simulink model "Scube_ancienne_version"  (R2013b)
settings: Solver=ode23t  StartTime=0.0  StopTime=100  RelTol=1e-3
libraries: fl_lib x14, nesl_utility x4, elec_lib x1

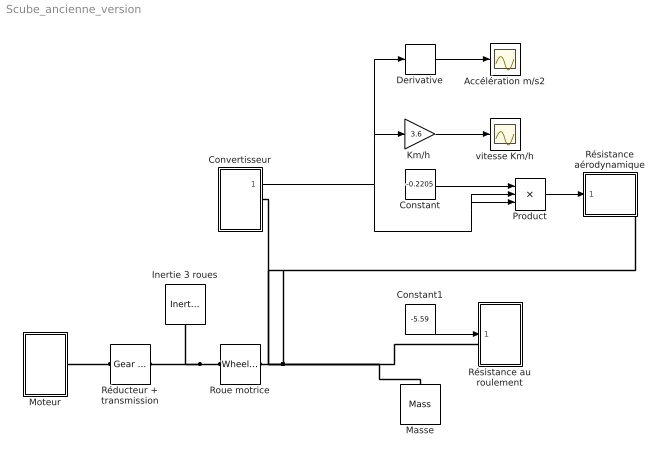
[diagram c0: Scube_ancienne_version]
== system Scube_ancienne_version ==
  Accélération m/s2 : Scope
  Constant : Constant  Value=-0.2205
  Constant1 : Constant  Value=-5.59
  Convertisseur : Subsystem
  Derivative : Derivative
  Inertie 3 roues : fl_lib/Mechanical/Rotational Elements/Inertia  inertia=0.01 kg*m^2  initial_velocity=0 rad/s  t_Log=off  LocalVarNames=|t  LocalVarDescs=|t  LocalVarLogging=0
  "Km/h " : Gain  Gain=3.6
  Masse : fl_lib/Mechanical/Translational Elements/Mass  mass=10 kg  initial_velocity=0 m/s  f_Log=off  LocalVarNames=|f  LocalVarDescs=|f  LocalVarLogging=0
  Moteur : Subsystem
  Product : Product  Inputs=3
  Roue motrice : fl_lib/Mechanical/Mechanisms/Wheel and Axle  R=50 mm  or=1  orient=1  t_Log=off  f_Log=off  LocalVarNames=|t|f  LocalVarDescs=|t|f  LocalVarLogging=[0 0]
  Réducteur + transmission : fl_lib/Mechanical/Mechanisms/Gear Box  ratio=13.84  t_in_Log=off  t_out_Log=off  LocalVarNames=|t_in|t_out  LocalVarDescs=|t_in|t_out  LocalVarLogging=[0 0]
  Résistance au roulement : Subsystem
  Résistance aérodynamique : Subsystem
  vitesse Km/h : Scope
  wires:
  "Km/h "/1 -> vitesse Km/h/1
  Constant1/1 -> Résistance au roulement/1(In1)
  Convertisseur/1(V (m/s)) -> Product/2, Product/3, Derivative/1, "Km/h "/1
  Constant/1 -> Product/1
  Product/1 -> Résistance aérodynamique/1(In1)
  Derivative/1 -> Accélération m/s2/1
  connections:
  Roue motrice/RConn1 -- Résistance aérodynamique/RConn1 -- Convertisseur/RConn1 -- Résistance au roulement/LConn1 -- Masse/LConn1
  Roue motrice/LConn1 -- Inertie 3 roues/LConn1 -- Réducteur + transmission/RConn1
  Moteur/RConn1 -- Réducteur + transmission/LConn1

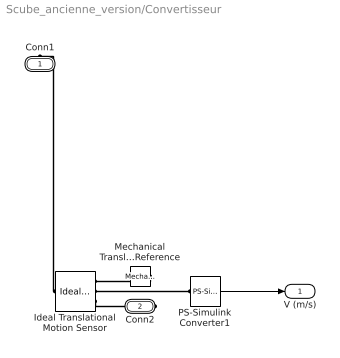
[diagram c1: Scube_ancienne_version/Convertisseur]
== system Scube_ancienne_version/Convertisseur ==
  Ideal Translational Motion Sensor : fl_lib/Mechanical/Mechanical Sensors/Ideal Translational Motion Sensor  offset=0 m  v_Log=off  f_Log=off  x_Log=off  LocalVarNames=|v|f|x  LocalVarDescs=|v|f|x  LocalVarLogging=[0 0 0]
  Mechanical Translational Reference : fl_lib/Mechanical/Translational Elements/Mechanical Translational Reference  f_Log=off  LocalVarNames=|f  LocalVarDescs=|f  LocalVarLogging=0
  PS-Simulink Converter1 : nesl_utility/PS-Simulink Converter  PhysicalDomain=network_engine_domain  SubClassName=ps_output  LeftPortType=input  RightPortType=output  PseudoPeriodic=off  Frequencies=[]  Unit=m/s  AffineConversion=off
  Conn1 : PMIOPort  Port=1  Side=Right
  Conn2 : PMIOPort  Port=2  Side=Right
  V (m/s) : Outport
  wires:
  PS-Simulink Converter1/1 -> V (m/s)/1
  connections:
  Ideal Translational Motion Sensor/RConn3 -- Conn2/RConn1
  Ideal Translational Motion Sensor/LConn1 -- Conn1/RConn1
  Mechanical Translational Reference/LConn1 -- Ideal Translational Motion Sensor/RConn1
  PS-Simulink Converter1/LConn1 -- Ideal Translational Motion Sensor/RConn2

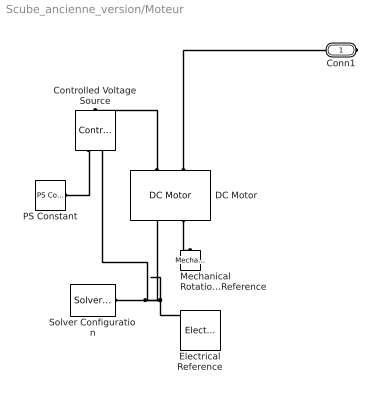
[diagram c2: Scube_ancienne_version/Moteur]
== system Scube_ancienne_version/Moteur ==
  Controlled Voltage Source : fl_lib/Electrical/Electrical Sources/Controlled Voltage Source  i_Log=off  v_Log=off  LocalVarNames=|i|v  LocalVarDescs=|i|v  LocalVarLogging=[0 0]
  DC Motor : elec_lib/Actuators & Drivers/Rotational Actuators/DC Motor  parameterization=2  Ra=2 Ohm  La=1 mH  emf_or_torque=2  Kv=4e-3 V/rpm  Ki=4e-2 N*m/A  T_stall=1.83333 N*m  w_max=3700 rpm  w_rated=3200 rpm  P_rated=600 W  V_rated=48 V  J=0.006 kg*m^2  lam_param=2  lam=0 N*m/(rad/s)  i_noload=2.2 A  V_i_noload=48 V  speed0=0 rpm  current_Log=off  voltage_Log=off  power_Log=off  i2r_Log=off  torque_Log=off  speed_Log=off  LocalVarNames=|current|voltage|power|i2r|torque|speed  LocalVarDescs=|Current (A)|Voltage (V)|Power (W)|Electrical losses (W)|Torque (Nm)|Angular speed (rad/s)  LocalVarLogging=[0 0 0 0 0 0]  alpha=0.00393 1/K  Tmeas=25 C  thermal_mass=100 J/K  initial_temperature=25 C
  Electrical Reference : fl_lib/Electrical/Electrical Elements/Electrical Reference  i_Log=off  LocalVarNames=|i  LocalVarDescs=|i  LocalVarLogging=0
  Mechanical Rotational Reference : fl_lib/Mechanical/Rotational Elements/Mechanical Rotational Reference  t_Log=off  LocalVarNames=|t  LocalVarDescs=|t  LocalVarLogging=0
  PS Constant : fl_lib/Physical Signals/Sources/PS Constant  constant=48  LocalVarLogging=[]
  Solver Configuration : nesl_utility/Solver Configuration  PhysicalDomain=network_engine_domain  SubClassName=solver  LeftPortType=input  RightPortType=generic  Accelerate=off  Tones=[]  Harmonics=[]  SimulateNoise=off  Profile=off  UseLocalSampling=off  EnableSwitchedLinearOptims=on  FrequencyDomain=off  UseCCode=off  RelTol=0.001  AbsTol=1e-06  MinStep=1e-09  ToWorkspace=off  DoDC=off  ResidualTolerance=1e-9  UseLocalSolver=off  LocalSolverChoice=NE_BACKWARD_EULER_ADVANCER  LocalSolverSampleTime=.001  DoFixedCost=off  MaxNonlinIter=3  MaxModeIter=2  LinearAlgebra=Sparse  DelaysMemoryBudget=1024
  Conn1 : PMIOPort  Port=1  Side=Right
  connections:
  Solver Configuration/RConn1 -- Electrical Reference/LConn1 -- Controlled Voltage Source/RConn2 -- DC Motor/RConn1
  DC Motor/LConn2 -- Conn1/RConn1
  DC Motor/RConn2 -- Mechanical Rotational Reference/LConn1
  Controlled Voltage Source/RConn1 -- PS Constant/RConn1
  DC Motor/LConn1 -- Controlled Voltage Source/LConn1

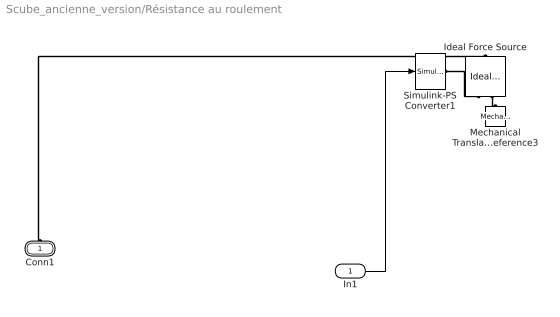
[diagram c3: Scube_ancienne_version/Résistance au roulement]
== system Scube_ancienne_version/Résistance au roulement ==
  In1 : Inport
  Ideal Force Source : fl_lib/Mechanical/Mechanical Sources/Ideal Force Source  v_Log=off  f_Log=off  LocalVarNames=|v|f  LocalVarDescs=|v|f  LocalVarLogging=[0 0]
  Mechanical Translational Reference3 : fl_lib/Mechanical/Translational Elements/Mechanical Translational Reference  f_Log=off  LocalVarNames=|f  LocalVarDescs=|f  LocalVarLogging=0
  Simulink-PS Converter1 : nesl_utility/Simulink-PS Converter  PhysicalDomain=network_engine_domain  SubClassName=ps_input  LeftPortType=input  RightPortType=output  PseudoPeriodic=off  Frequencies=[]  NoiseDistribution=none  NoiseParameters=[]  Unit=1  AffineConversion=off  InputFiltering=off  SimscapeFilterOrder=1  InputFilterTimeConstant=0.001  UdotUserProvided=1
  Conn1 : PMIOPort  Port=1  Side=Left
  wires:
  In1/1 -> Simulink-PS Converter1/1
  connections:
  Ideal Force Source/RConn1 -- Simulink-PS Converter1/RConn1
  Ideal Force Source/RConn2 -- Mechanical Translational Reference3/LConn1
  Ideal Force Source/LConn1 -- Conn1/RConn1

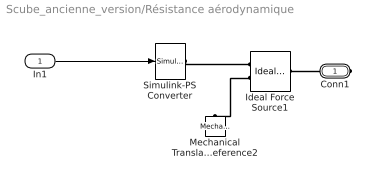
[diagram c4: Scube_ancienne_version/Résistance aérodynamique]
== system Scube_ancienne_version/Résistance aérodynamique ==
  In1 : Inport
  Ideal Force Source1 : fl_lib/Mechanical/Mechanical Sources/Ideal Force Source  v_Log=off  f_Log=off  LocalVarNames=|v|f  LocalVarDescs=|v|f  LocalVarLogging=[0 0]
  Mechanical Translational Reference2 : fl_lib/Mechanical/Translational Elements/Mechanical Translational Reference  f_Log=off  LocalVarNames=|f  LocalVarDescs=|f  LocalVarLogging=0
  Simulink-PS Converter : nesl_utility/Simulink-PS Converter  PhysicalDomain=network_engine_domain  SubClassName=ps_input  LeftPortType=input  RightPortType=output  PseudoPeriodic=off  Frequencies=[]  NoiseDistribution=none  NoiseParameters=[]  Unit=1  AffineConversion=off  InputFiltering=off  SimscapeFilterOrder=1  InputFilterTimeConstant=0.001  UdotUserProvided=1
  Conn1 : PMIOPort  Port=1  Side=Right
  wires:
  In1/1 -> Simulink-PS Converter/1
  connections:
  Simulink-PS Converter/RConn1 -- Ideal Force Source1/RConn1
  Ideal Force Source1/RConn2 -- Mechanical Translational Reference2/LConn1
  Ideal Force Source1/LConn1 -- Conn1/RConn1
